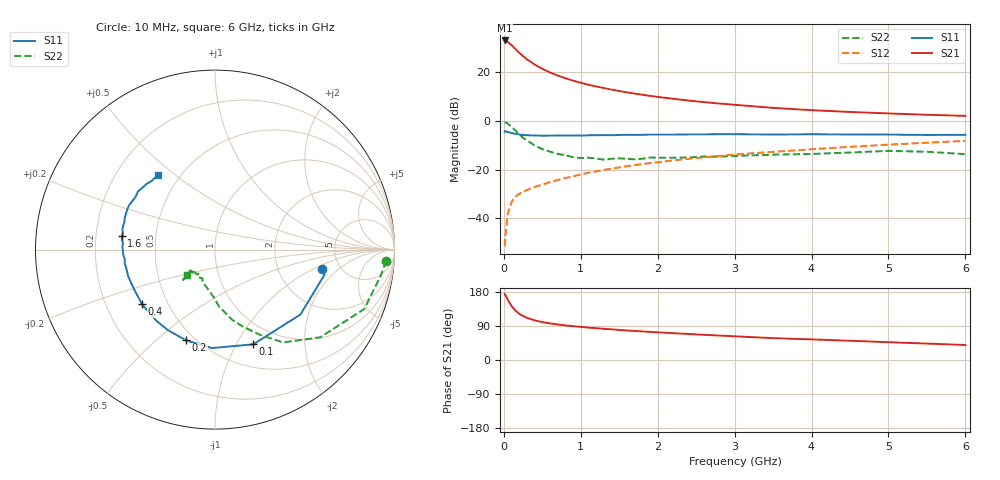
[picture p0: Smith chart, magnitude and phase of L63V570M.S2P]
!  INFINEON TECHNOLOGIES Small Signal Semiconductors
! BFR380L3 , Si-NPN RF-Transistor in TSLP-3-1
!  Vce=3.5 V,  Ic=70 mA
! Common Emitter S-Parameters:  07. March 2005
#  GHz  S  MA  R  50
! f  S11  S21  S12  S22
! GHz  Mag  Ang  Mag  Ang  Mag  Ang  Mag  Ang
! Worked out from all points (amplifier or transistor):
!   36 points, 10 MHz to 6 GHz, reference 50 ohm
!   highest |S21| = 33.1 dB at 10 MHz (marker M1)
!   |S21| within 3 dB of that: start of sweep to 134.2 MHz
!   unconditionally stable (mu >= 1): 1.337 GHz to 4.819 GHz
!   at 250 MHz: K = 0.52, MSG = 27.9 dB, |S12| = -29.1 dB
!   at 1.4 GHz: K = 1.01, MAG = 15.7 dB, |S12| = -19.6 dB
!   at 6 GHz: K = 0.97, MSG = 5.1 dB, |S12| = -8.1 dB
!   S11 on the Smith chart (normalised r, x): 10 MHz: 3.60, -1.23; 100 MHz: 0.75, -1.18; 200 MHz: 0.45, -0.63; 400 MHz: 0.36, -0.29; 1.6 GHz: 0.31, +0.06; 6 GHz: 0.38, +0.43
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0.01  0.604 -10.3  45.44 174.0  0.0027 78.3  0.9551 -3.8
0.02  0.6263 -12.9  45.27 171.6  0.0043 86.7  0.936 -8.7
0.05  0.5977 -37.3  42.65 159.2  0.0123 76.6  0.8949 -21.7
0.1  0.5693 -68.0  36.48 142.6  0.0217 64.9  0.7633 -39.8
0.15  0.5489 -91.8  30.36 130.4  0.0279 58.4  0.6417 -53.7
0.2  0.5307 -107.7  25.38 122.0  0.032 56.1  0.5391 -62.0
0.25  0.5199 -120.3  21.62 116.0  0.035 54.7  0.4542 -70.3
0.3  0.5136 -129.6  18.61 111.3  0.0384 54.9  0.4039 -76.1
0.4  0.5079 -143.1  14.55 104.6  0.0445 55.3  0.3172 -86.1
0.5  0.5017 -152.1  11.9 100.1  0.0496 58.3  0.2656 -91.3
0.6  0.5032 -158.5  9.979 96.6  0.0559 59.9  0.236 -97.3
0.7  0.5061 -163.2  8.646 93.8  0.0617 61.2  0.2128 -103.2
0.9  0.509 -171.7  6.776 89.3  0.0734 64.0  0.1825 -113.0
1.1  0.512 -176.8  5.601 85.5  0.0871 65.7  0.178 -118.0
1.3  0.5161 177.9  4.781 82.2  0.0999 66.6  0.1618 -125.3
1.6  0.5245 171.9  3.9 77.9  0.1186 67.1  0.168 -132.6
2.2  0.528 163.0  2.878 70.7  0.1558 67.3  0.1771 -134.0
2.8  0.5384 154.6  2.3 64.5  0.1927 67.1  0.1865 -139.8
3.5  0.5312 146.3  1.873 57.7  0.234 64.7  0.205 -138.0
4.5  0.5325 140.4  1.544 50.8  0.2968 63.0  0.2267 -137.1
5.5  0.5203 132.3  1.352 43.3  0.3604 59.0  0.2348 -136.6
6  0.5233 127.5  1.282 39.6  0.3931 56.8  0.21 -138.6
